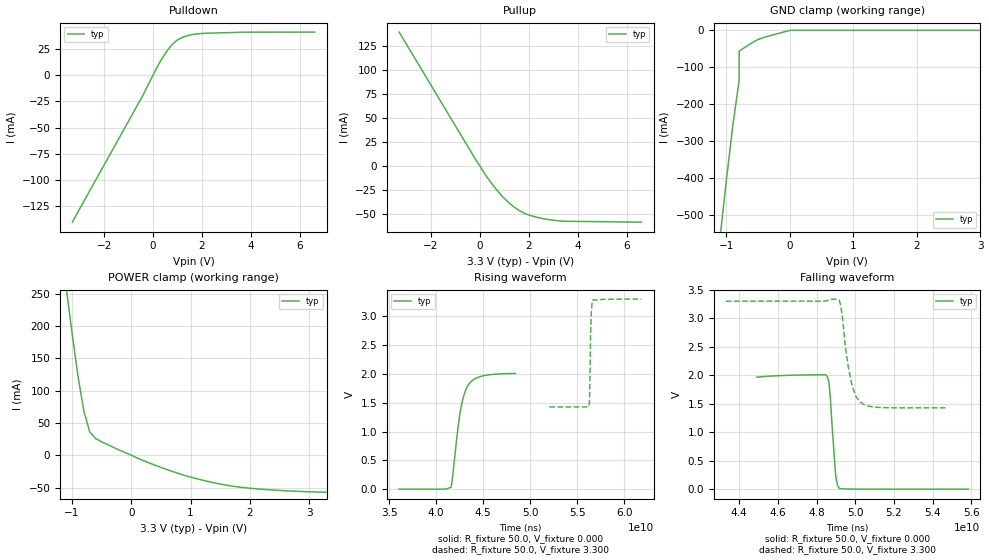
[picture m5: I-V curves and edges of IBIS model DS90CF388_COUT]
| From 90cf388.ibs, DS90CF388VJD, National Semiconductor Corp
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|   CLK Output  MODEL
[Model]   DS90CF388_COUT
Model_type   Output
| Signals
Vmeas = 1.5V
Cref = 8pF   |Timing specification test load capacitance value
Rref = 50.0
Vref = 0.0   |Timing specification test load voltage; GND
Vinl = 0.8
Vinh = 2.0
| variable   typ   min   max
C_comp   5.753pF   NA   NA
|   typ   min   max
[Temperature Range]   25.0   -10   70
[Voltage range]   3.3V   3.0V   3.6V
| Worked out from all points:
|   slope of the pulldown table from 0 to 0.495 V, typ, clamps not added: 24.3 ohm
|   slope of the pullup table from 0 to 0.495 V, typ, clamps not added: 26.3 ohm
|   GND clamp passes 1 mA (typ) near -0.02 V on its own axis
|   POWER clamp passes 1 mA (typ) near -0.01 V on its own axis
|   falling waveform, R_fixture 50.0, V_fixture 0.000: 20-80 % time 236ms typ, NA min, NA max; typ from 1.97 V to 0 V
|   falling waveform, R_fixture 50.0, V_fixture 3.300: 20-80 % time 482ms typ, NA min, NA max; typ from 3.3 V to 1.43 V
|   rising waveform, R_fixture 50.0, V_fixture 0.000: 20-80 % time 1.04s typ, NA min, NA max; typ from 0 V to 2.01 V
|   rising waveform, R_fixture 50.0, V_fixture 3.300: 20-80 % time 128ms typ, NA min, NA max; typ from 1.43 V to 3.3 V
[Pulldown]
| Voltage   I(typ)   I(min)   I(max)
-3.3V     -140mA     NA         NA
-400mV    -18.74mA   NA         NA
300mV     13.25mA    NA         NA
600mV     23.82mA    NA         NA
900mV     31.54mA    NA         NA
1.1V      34.72mA    NA         NA
1.3V      36.56mA    NA         NA
1.6V      38.36mA    NA         NA
2V        39.47mA    NA         NA
3.6V      40.66mA    NA         NA
6.6V      40.76mA    NA         NA
[Pullup]
| Note that the[Pullup]voltage table is referenced to Vcc
| and is calculated using Vtable=Vcc - Vmeasured.
|Voltage   I(typ)   I(min)   I(max)
-3.3V     140mA      NA         NA
100mV     -3.97mA    NA         NA
500mV     -18.51mA   NA         NA
900mV     -31.04mA   NA         NA
1.3V      -40.48mA   NA         NA
1.6V      -45.94mA   NA         NA
1.9V      -49.8mA    NA         NA
2.4V      -53.57mA   NA         NA
2.9V      -55.89mA   NA         NA
3.4V      -57.25mA   NA         NA
6.6V      -58.25mA   NA         NA
[GND_clamp]
| Outputs in Tri-state.
| Voltage   I(typ)   I(min)   I(max)
-3.3V     -4.304A    NA         NA
-1.1V     -560mA     NA         NA
-1V       -403.9mA   NA         NA
-900mV    -258mA     NA         NA
-800mV    -134.5mA   NA         NA
-500mV    -24.5mA    NA         NA
0V        -48.52uA   NA         NA
3V        0A         NA         NA
[POWER_clamp]
| Note that the[POWER_clamp]voltage table is referenced to Vcc
| and is calculated using Vtable=Vcc - Vmeasured.
| Outputs in Tri-state.
|Voltage   I(typ)   I(min)   I(max)
-3.3V     1.984A     NA         NA
-1.1V     261.5mA    NA         NA
-1V       189.8mA    NA         NA
-900mV    123.2mA    NA         NA
-800mV    68.63mA    NA         NA
-700mV    36.18mA    NA         NA
-600mV    25.97mA    NA         NA
400mV     -15.08mA   NA         NA
900mV     -31.04mA   NA         NA
1.3V      -40.48mA   NA         NA
2V        -50.71mA   NA         NA
3.3V      -57.03mA   NA         NA
[Ramp]
|   typ   min   max
dV/dt_r   1.023/1.17n   NA   NA
dV/dt_f   1.006/0.41n   NA   NA
R_load = 50Ohm
[Falling Waveform]
R_fixture = 50.0
V_fixture = 0.000
C_fixture = 0.0pF
| Time   V(typ)   V(min)   V(max)
44.92s    1.965V     NA         NA
48.4s     2.009V     NA         NA
48.56s    1.974V     NA         NA
48.64s    1.878V     NA         NA
48.71s    1.626V     NA         NA
48.79s    1.187V     NA         NA
48.99s    236.7mV    NA         NA
49.08s    70.2mV     NA         NA
49.18s    13.13mV    NA         NA
55.84s    21.93uV    NA         NA
[Falling Waveform]
R_fixture = 50.0
V_fixture = 3.300
C_fixture = 0.0pF
|  Time   V(typ)   V(min)   V(max)
43.32s    3.298V     NA         NA
49.17s    3.318V     NA         NA
49.32s    3.072V     NA         NA
49.48s    2.524V     NA         NA
49.65s    2.126V     NA         NA
49.85s    1.8V       NA         NA
50.05s    1.618V     NA         NA
50.25s    1.53V      NA         NA
51.25s    1.434V     NA         NA
54.65s    1.428V     NA         NA
[Rising Waveform]
R_fixture = 50.0
V_fixture = 0.000
C_fixture = 0.0pF
| Time   V(typ)   V(min)   V(max)
36.05s    51.62uV    NA         NA
41.58s    33.02mV    NA         NA
41.79s    276.5mV    NA         NA
42.32s    1.072V     NA         NA
42.52s    1.307V     NA         NA
42.92s    1.615V     NA         NA
43.32s    1.785V     NA         NA
43.92s    1.896V     NA         NA
44.92s    1.965V     NA         NA
48.42s    2.009V     NA         NA
[Rising Waveform]
R_fixture = 50.0
V_fixture = 3.300
C_fixture = 0.0pF
| Time   V(typ)   V(min)   V(max)
52.05s    1.428V     NA         NA
56.17s    1.425V     NA         NA
56.3s     1.473V     NA         NA
56.34s    1.706V     NA         NA
56.37s    1.987V     NA         NA
56.43s    2.676V     NA         NA
56.49s    3.003V     NA         NA
56.57s    3.206V     NA         NA
56.7s     3.285V     NA         NA
61.85s    3.3V       NA         NA
